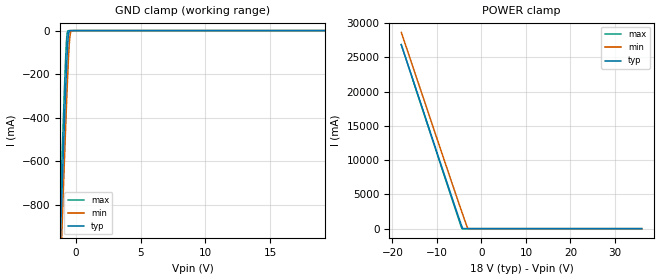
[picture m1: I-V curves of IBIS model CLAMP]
| Texas Instruments Incorporated
| TVS1800 18-V FlatClamp Surge Protection Device
[IBIS Ver]   4.1
[File name]   tvs1800.ibs
[File Rev]   1.0
[Date]   12/15/2017
[Source]
| Texas Instruments Incorporated.
| Analog-eLab Design Center, HPA
| 12500 TI Blvd
| Dallas, TX -75243
[Notes]   Revision History:
| Rev 1.0: 12/15/2017
| - Initial version of the model
| - Model generated from simulations in SPECTRE
| - Model matched to SPICE simulation
| - C_comp although listed in numerical order of value are
|   obtained from varying PVT conditions. For PVT conditions for
|   each specific value refer the buffer description under
|   respective [Model]. IBIS model user is responsible for using
|   appropriate C_comp to simulate for Signal Integrity.
[Disclaimer]
| This model is designed as an aid for customers of Texas Instruments.
| TI and its licensors and suppliers make no warranties, either expressed
| or implied, with respect to this  model, including the warranties of
| merchantability or fitness for a particular purpose. The model is
| provided solely on an "as is" basis. The entire risk as to its quality
| and performance is with the customer.
[Copyright]
(C) Copyright 2017 Texas Instruments Incorporated.All rights reserved.
|   TVS1800
[Component]   TVS1800DRV
[Manufacturer]   TI
[Package]   |6-pin SON DRV package
|   typ   min   max
R_pkg   0.03312   0.03141   0.03462
L_pkg   0.49614nH   0.44882nH   0.53669nH
C_pkg   0.15951pF   0.15201pF   0.17090pF
[Pin]  signal_name model_name   R_pin   L_pin  C_pin
1   GND   GND   NA   NA   NA
2   GND   GND   NA   NA   NA
3   GND   GND   NA   NA   NA
4   IN   CLAMP   NA   NA   NA
5   IN   CLAMP   NA   NA   NA
6   IN   CLAMP   NA   NA   NA
| Models and submodels in the file (1): CLAMP (Terminator)
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|   Model CLAMP
[Model]   CLAMP
Model_type   Terminator
|   typ   min   max
C_comp   8.465E-11  8.122E-11   8.504E-11
|Where Nom  PVT is Nominal Process, 18V,   40C
|   Fast PVT is Strong Process,  18.001V, -40C
|   Slow PVT is Weak Process,   17.999V, 125C
[Voltage Range]   18   17.999   18.001
[Temperature Range]   40   125   -40
[Power Clamp Reference]   18   17.999   18.001
[GND Clamp Reference]   0   0   0
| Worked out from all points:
|   GND clamp passes 1 mA (typ) near -0.46 V on its own axis
|   POWER clamp passes 1 mA (typ) near -4.13 V on its own axis
[GND Clamp]
|   Voltage   I(typ)   I(min)   I(max)
-18V      -33.24A    -33.24A    -33.27A
-1.26V    -1.089A    -1.262A    -935.8mA
-1.152V   -901.3mA   -1.075A    -746.7mA
-1.044V   -715.4mA   -889.3mA   -560mA
-828mV    -355.8mA   -527.6mA   -203.6mA
-720mV    -190.3mA   -355.6mA   -55.65mA
-666mV    -116.5mA   -273.7mA   -13.23mA
-558mV    -16.87mA   -126.2mA   -321.2uA
-450mV    -485.4uA   -27.38mA   -27.07uA
-396mV    -53.2uA    -8.063mA   0A
-126mV    0A         0A         0A
36V       0A         0A         0A
[POWER Clamp]
|   Voltage   I(typ)   I(min)   I(max)
-18V      26.85A     28.63A     26.82A
-4.554V   602.1mA    2.721A     311mA
-4.392V   308.7mA    2.417A     34.9mA
-4.176V   5.413mA    2.012A     139.2uA
-3.042V   0A         31.68mA    0A
36V       0A         0A         0A
